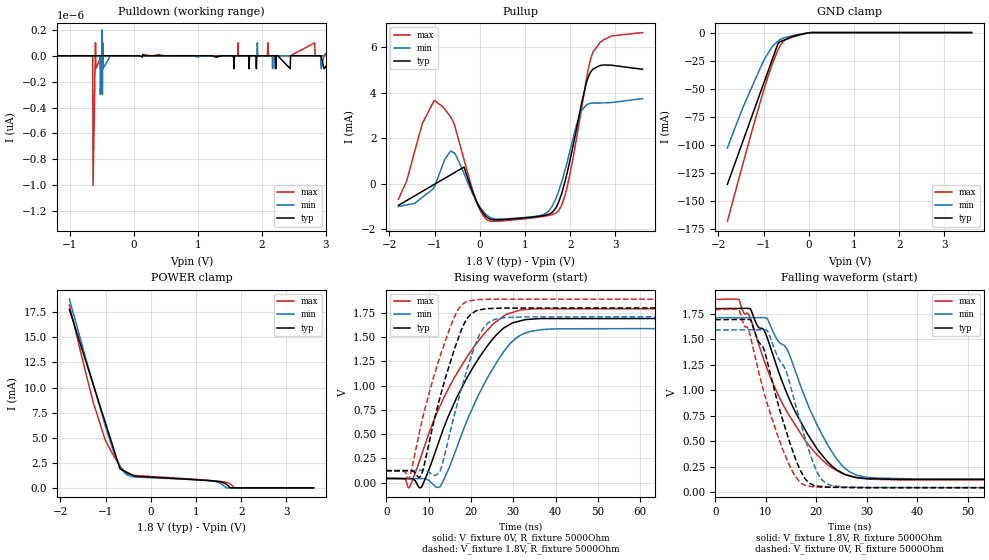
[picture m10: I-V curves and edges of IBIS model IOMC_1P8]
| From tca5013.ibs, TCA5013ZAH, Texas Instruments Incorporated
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|   Model IOMC
[Model]   IOMC_1P8
Model_type   I/O
Polarity   Non-Inverting
Enable   Active-Low
Vinl = .54
Vinh = 1.26
Vmeas = 0.9
Vref = 1.8
Cref = 1pF
Rref = 5000
|   typ   min   max
C_comp   0.597p   0.445p   0.907p
|C_comp (ON state)   0.597p   0.445p   0.907p
|C_comp (OFF state)   0.592p   0.445p   0.907p
[Model spec]
|subparameter
Vinl   0.54   0.513   0.567
Vinh   1.26   1.197   1.323
[Voltage Range]   1.8   1.71   1.89
[Temperature Range]   27   125   -40
[Pullup Reference]   1.8   1.71   1.89
[Pulldown Reference]   0   0   0
[Power Clamp Reference]   1.8   1.71   1.89
[GND Clamp Reference]   0   0   0
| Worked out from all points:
|   slope of the pullup table from 0 to 0.27 V, typ, clamps not added: 527 ohm
|   GND clamp passes 1 mA (typ) near -0.10 V on its own axis
|   falling waveform, V_fixture 1.8V, R_fixture 5000Ohm: 20-80 % time 9.09ns typ, 8.22ns min, 10.2ns max; typ from 1.8 V to 0.122 V
|   rising waveform, V_fixture 0V, R_fixture 5000Ohm: 20-80 % time 11.1ns typ, 10.1ns min, 12.3ns max; typ from 0.043 V to 1.69 V
|   rising waveform, V_fixture 1.8V, R_fixture 5000Ohm: 20-80 % time 6.47ns typ, 6.11ns min, 6.94ns max; typ from 0.122 V to 1.8 V
|   falling waveform, V_fixture 0V, R_fixture 5000Ohm: 20-80 % time 5.69ns typ, 6.04ns min, 6.22ns max; typ from 1.69 V to 0.043 V
[Pulldown]
|   Voltage   I(typ)   I(min)   I(max)
-1.8V     0A         0A         0A
-1.789V   0A         -10pA      0A
-1.784V   0A         0A         0A
-1.735V   0A         -1pA       0A
-1.606V   0A         0A         0A
-644.4mV  0A         0A         0A
-639mV    0A         0A         -1pA
-601.2mV  0A         0A         100fA
3.438V    0A         0A         0A
3.443V    -1pA       0A         0A
3.449V    0A         0A         0A
3.6V      0A         0A         0A
[GND Clamp]
|   Voltage   I(typ)   I(min)   I(max)
-1.8V     -135.3mA   -102.9mA   -168.2mA
-1.438V   -94.7mA    -64.94mA   -114.3mA
-1.271V   -75.93mA   -49.7mA    -89.73mA
-1.025V   -48.33mA   -27.31mA   -55.18mA
-936mV    -38.38mA   -20.67mA   -43.39mA
-821.3mV  -25.51mA   -13.39mA   -29.59mA
-682.2mV  -9.917mA   -7.743mA   -15.53mA
-601.2mV  -7.629mA   -5.624mA   -9.831mA
-541.8mV  -6.608mA   -4.639mA   -7.271mA
-347.4mV  -3.267mA   -2.721mA   -3.958mA
52.2mV    0A         0A         0A
3.6V      0A         0A         0A
[Pullup]
|   Voltage   I(typ)   I(min)   I(max)
-1.8V     -952.7uA   -1.004mA   -682.5uA
-1.271V   -337.6uA   -599.3uA   2.645mA
-1.01V    -34.04uA   -161.5uA   3.657mA
-644.4mV  390.4uA    1.44mA     2.941mA
-347.4mV  735.6uA    444uA      1.054mA
160.2mV   -1.476mA   -1.385mA   -1.585mA
1.37V     -1.416mA   -1.382mA   -1.448mA
1.694V    -1.024mA   -600.2uA   -1.276mA
1.921V    379.4uA    862.8uA    -239.5uA
2.207V    3.085mA    3.003mA    2.772mA
2.509V    5.045mA    3.547mA    5.804mA
3.6V      5.031mA    3.745mA    6.645mA
[POWER Clamp]
|   Voltage   I(typ)   I(min)   I(max)
-1.8V     17.78mA    18.81mA    18.22mA
-1.271V   10.27mA    10.29mA    8.489mA
-1.01V    6.559mA    6.234mA    4.797mA
-806.4mV  3.674mA    3.425mA    3.085mA
-682.2mV  1.911mA    2.183mA    2.199mA
-563.4mV  1.631mA    1.425mA    1.551mA
-347.4mV  1.15mA     1.098mA    1.238mA
1.51V     622.6uA    509.6uA    657.4uA
1.661V    387.3uA    19.99uA    556.7uA
1.764V    0A         0A         364.1uA
1.85V     0A         0A         0A
3.6V      0A         0A         0A
[Ramp]
R_load = 5000
|   typ   min   max
dV/dt_r   0.989086/1.10693e-08   0.928638/1.00678e-08   1.04797/1.22586e-08
dV/dt_f   1.00653/9.05178e-09   0.950591/8.1991e-09   1.0601/1.0241e-08
[Falling Waveform]
V_fixture = 1.8V
V_fixture_min = 1.71V
V_fixture_max = 1.89V
R_fixture = 5000Ohm
C_fixture = 0F
|   Time   V(typ)   V(min)   V(max)
0s        1.8V       1.71V      1.89V
4.734ns   1.802V     1.711V     1.886V
7.018ns   1.795V     1.711V     1.7V
10.32ns   1.513V     1.704V     1.207V
12.19ns   1.236V     1.502V     985.1mV
14.36ns   949.5mV    1.388V     776.7mV
18.2ns    578.3mV    879.9mV    484.9mV
25.18ns   189.2mV    259.2mV    180.7mV
31.87ns   130.7mV    138.8mV    125.4mV
99.9ns    122.3mV    125.4mV    123mV
[Rising Waveform]
V_fixture = 0V
V_fixture_min = 0V
V_fixture_max = 0V
R_fixture = 5000Ohm
C_fixture = 0F
|   Time   V(typ)   V(min)   V(max)
0s        42.67mV    42.49mV    43.99mV
4.235ns   40.98mV    41.77mV    41.68mV
5.448ns   40.5mV     41.57mV    -51.87mV
8.269ns   -50mV      41.09mV    275.2mV
12.69ns   454.2mV    -43.17mV   787.5mV
19.12ns   1.085V     642.5mV    1.297V
28.28ns   1.606V     1.379V     1.732V
31.87ns   1.668V     1.522V     1.779V
36.72ns   1.689V     1.576V     1.791V
99.9ns    1.691V     1.59V      1.791V
[Rising Waveform]
V_fixture = 1.8V
V_fixture_min = 1.71V
V_fixture_max = 1.89V
R_fixture = 5000Ohm
C_fixture = 0F
|   Time   V(typ)   V(min)   V(max)
0s        122.1mV    125.2mV    123mV
4.194ns   121.9mV    125.1mV    120.9mV
5.448ns   121.8mV    125mV      48.37mV
8.269ns   74.85mV    124.9mV    601.2mV
12.69ns   877.1mV    117.7mV    1.295V
16.43ns   1.415V     753.1mV    1.738V
19.01ns   1.684V     1.155V     1.865V
22.93ns   1.786V     1.593V     1.887V
28.04ns   1.798V     1.7V       1.889V
99.9ns    1.8V       1.71V      1.89V
[Falling Waveform]
|Gnd
V_fixture = 0V
V_fixture_min = 0V
V_fixture_max = 0V
R_fixture = 5000Ohm
C_fixture = 0F
|   Time   V(typ)   V(min)   V(max)
0s        1.691V     1.59V      1.791V
4.768ns   1.693V     1.591V     1.784V
7.095ns   1.681V     1.592V     1.501V
10.42ns   1.261V     1.577V     850.3mV
14.61ns   513.2mV    1.098V     274.1mV
17.87ns   128.9mV    520.4mV    66.61mV
19.74ns   63.21mV    246.6mV    51.95mV
21.14ns   54.89mV    122mV      49.34mV
25.3ns    47.2mV     50.88mV    46.62mV
99.9ns    42.68mV    42.5mV     43.99mV
